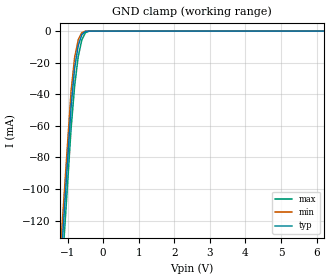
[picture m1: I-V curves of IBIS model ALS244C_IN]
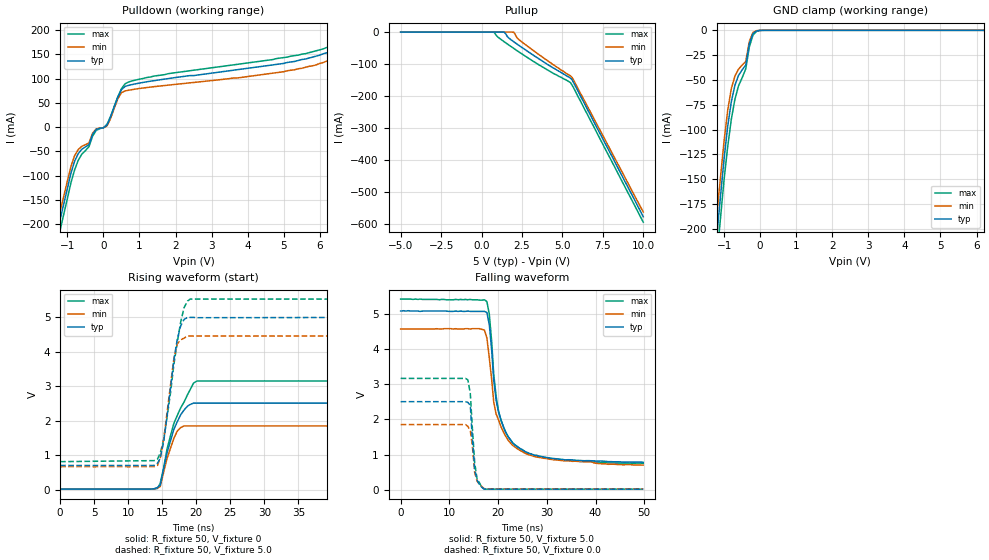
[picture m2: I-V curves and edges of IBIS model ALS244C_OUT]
| TEXAS INSTRUMENTS INCORPORATED
| Standard Linear and Logic Group
| IBIS Model of SN74ALS244C
| OCTAL BUFFERS AND LINE DRIVERS WITH 3-STATE OUTPUTS
| SOIC 20-pin (DW), SOP 20-pin (NS), SSOP 20-pin (DB), PDIP 20-pin (N) Package
[IBIS Ver]   3.2
[Comment Char]  |_char
[File Name]   sn54als244cw.ibs
[File Rev]   3.1
[Date]   Sept. 23, 2004
[Source]   Data created from Labo data at TI-SLL.
[Notes]   The following is an IBIS list for the ALS244C.
   - FILE REV HISTORY
   - 3.1 Re-Release IBIS file on 09/23/04
   - Power clamp data deleted as there is no power-clamp diode
|   Please contact sllibis@ti.com with questions and
|   comments concerning SLL IBIS models.
|   Modified for W ceramice package.  01/14/2009
[Disclaimer] Property of Texas Instruments Incorporated.  Unauthorized
   reproduction and/or distribution is strictly prohibited.
   This product is protected under copyright law.
   Created 2000, (C) Copyright 2000, Texas Instruments Inc.,
   All Rights Reserved.
   UNLESS THERE IS A SIGNED, WRITTEN AGREEMENT TO THE
   CONTRARY, TEXAS INSTRUMENTS () IS PROVIDING THE IBIS
   MODELS  AND WITHOUT ANY WARRANTY, EXPRESSED OR
   IMPLIED.  TI assumes no liability for:
   1) the accuracy of the IBIS models provided to your
   company;
   2) the proper functioning of these IBIS Models in your
   design or for any resulting applications; or
   3) infringement of patents, copyrights or intellectual
   property rights resulting from your use of these IBIS
   models.
   TI provides IBIS Models as a service to our customers.
   You and your company shall not distribute, sell or give
   these models to anyone else without prior written
   permission from TI.
   TI reserves the right to make changes to our products or
   to discontinue any semiconductor product or service
   without notice, and advises our customers to obtain the
   latest version of relevant information to verify, before
   placing orders, that the information being relied on is
   current.
   Please be aware that your receipt and use of the IBIS
   information provided shall serve as acceptance of these
   terms and conditions.  If you do not accept these terms,
   you should return or destroy the IBIS models and any
   other accompanying information immediately.
|   Component ALS244C_W
[Component]   ALS244C_W
[Manufacturer]  Texas Instruments, Inc.
[Package]
|   typ   min   max
R_pkg   0.134   0.093   0.180
L_pkg   6.136nH   4.282nH   8.371nH
C_pkg   1.657pF   1.224pF   2.253pF
[Pin]   signal_name   model_name   R_pin   L_pin   C_pin
1   1OE_NOT   ALS244C_IN   0.161   8.173nH   2.244pF
2   1A1   ALS244C_IN   0.163   7.152nH   2.034pF
3   2Y4   ALS244C_OUT   0.154   6.346nH   1.604pF
4   1A2   ALS244C_IN   0.093   4.737nH   1.272pF
5   2Y3   ALS244C_OUT   0.097   4.297nH   1.227pF
6   1A3   ALS244C_IN   0.096   4.289nH   1.226pF
7   2Y2   ALS244C_OUT   0.093   4.759nH   1.269pF
8   1A4   ALS244C_IN   0.143   6.181nH   1.554pF
9   2Y1   ALS244C_OUT   0.164   7.085nH   1.905pF
10   GND   GND   0.175   8.294nH   2.233pF
11   2A1   ALS244C_IN   0.180   8.371nH   2.239pF
12   1Y4   ALS244C_OUT   0.155   7.195nH   1.934pF
13   2A2   ALS244C_IN   0.154   6.339nH   1.581pF
14   1Y3   ALS244C_OUT   0.096   4.872nH   1.281pF
15   2A3   ALS244C_IN   0.097   4.338nH   1.233pF
16   1Y2   ALS244C_OUT   0.097   4.282nH   1.224pF
17   2A4   ALS244C_IN   0.093   4.726nH   1.262pF
18   1Y1   ALS244C_OUT   0.143   6.164nH   1.571pF
19   2OE_NOT   ALS244C_IN   0.159   6.938nH   2.001pF
20   VCC   POWER   0.166   8.186nH   2.253pF
| Models and submodels in the file (2): ALS244C_IN (Input), ALS244C_OUT (3-state)
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|   Model ALS244C_IN
[Model]   ALS244C_IN
Model_type  Input
Polarity   Non-Inverting
Vinl = 0.8
Vinh = 2.0
| variable   typ   min   max
C_comp   1.33pf   1.00pf   1.66pf
[Temperature Range]   25   0   70
[Voltage Range]   5.0   4.5   5.5
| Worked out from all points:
|   GND clamp passes 1 mA (typ) near -0.54 V on its own axis
[GND Clamp]
|   Voltage   I(typ)   I(min)   I(max)
-5V       -1.46A     -1.41A     -1.52A
-1.2V     -151mA     -138mA     -168mA
-1.1V     -117mA     -105mA     -132mA
-1V       -82.2mA    -71.2mA    -96.9mA
-900mV    -47.7mA    -37.7mA    -61.4mA
-800mV    -23.3mA    -16.5mA    -34.4mA
-700mV    -9.09mA    -5.49mA    -16.1mA
-600mV    -2.32mA    -965uA     -5.65mA
-500mV    -207uA     -49.9uA    -1.1mA
-400mV    -20.2uA    -16uA      -84.4uA
-300mV    -13.8uA    -14.7uA    -15.1uA
10V       2.13nA     225pA      4.62nA
|   Model ALS244C_OUT
[Model]   ALS244C_OUT
Model_type  3-state
Polarity   Non-Inverting
Enable   Active-Low
Vmeas = 2.5v
Cref = 15pf
| variable   typ   min   max
C_comp   5.8pf   4.35pf   7.25pf
[Temperature Range]   25   0   70
[Voltage Range]   5.0   4.5   5.5
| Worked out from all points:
|   slope of the pulldown table from 0 to 0.75 V, typ, clamps not added: 8.52 ohm
|   GND clamp passes 1 mA (typ) near -0.11 V on its own axis
|   rising waveform, R_fixture 50, V_fixture 0: 20-80 % time 2.21ns typ, 1.63ns min, 2.94ns max; typ from 0.021 V to 2.51 V
|   falling waveform, R_fixture 50, V_fixture 5.0: 20-80 % time 3.03ns typ, 3.61ns min, 2.9ns max; typ from 5.07 V to 0.782 V
|   rising waveform, R_fixture 50, V_fixture 5.0: 20-80 % time 1.7ns typ, 1.46ns min, 2.03ns max; typ from 0.706 V to 4.99 V
|   falling waveform, R_fixture 50, V_fixture 0.0: 20-80 % time 832ps typ, 914ps min, 943ps max; typ from 2.5 V to 0.019 V
[Pulldown]
|   Voltage   I(typ)   I(min)   I(max)
-5V       -1.4A      -1.34A     -1.44A
-1.4V     -254mA     -234mA     -276mA
-1.2V     -190mA     -173mA     -212mA
-900mV    -94.5mA    -80.4mA    -114mA
-700mV    -54.5mA    -46.1mA    -68.4mA
-200mV    -4.82mA    -3.55mA    -6.79mA
100mV     4.21mA     2.48mA     5.91mA
500mV     76.9mA     70.9mA     79.1mA
700mV     86mA       75.9mA     92.9mA
5.8V      144mA      126mA      155mA
7.6V      239mA      228mA      252mA
10V       425mA      436mA      450mA
[Pullup]
|   Voltage   I(typ)   I(min)   I(max)
-5V       18.8nA     1.71nA     273nA
700mV     18.8nA     1.71nA     -78.4uA
800mV     18.8nA     1.71nA     -1.62mA
1V        18.8nA     1.71nA     -15mA
1.4V      -389uA     1.71nA     -30.2mA
1.6V      -14.4mA    1.69nA     -37.3mA
2V        -30.5mA    -634uA     -51.3mA
2.2V      -37.6mA    -18.3mA    -58.2mA
2.6V      -51.7mA    -35mA      -71.7mA
5.5V      -144mA     -137mA     -158mA
5.7V      -159mA     -151mA     -175mA
10V       -578mA     -563mA     -595mA
[GND Clamp]
|   Voltage   I(typ)   I(min)   I(max)
-5V       -1.67A     -1.58A     -1.72A
-1.3V     -245mA     -222mA     -268mA
-1.2V     -206mA     -185mA     -228mA
-1.1V     -167mA     -148mA     -189mA
-900mV    -96.5mA    -80.3mA    -117mA
-800mV    -71.9mA    -58.7mA    -89.6mA
-600mV    -45.4mA    -39.1mA    -55.9mA
-400mV    -35mA      -31.3mA    -38.8mA
-300mV    -13.4mA    -11.1mA    -16.7mA
-200mV    -3.29mA    -2.13mA    -4.83mA
-100mV    -596uA     -308uA     -1.06mA
10V       3.02nA     210pA      25.3nA
[Ramp]
| variable   typ   min   max
dV/dt_r   1.52E+00/2.32E-09   1.31E+00/2.29E-09   1.70E+00/2.40E-09
dV/dt_f   2.63E+00/3.12E-09   2.33E+00/3.42E-09   2.86E+00/2.98E-09
R_load = 50
[Rising Waveform]
R_fixture = 50
V_fixture = 0
|   Time   V(typ)   V(min)   V(max)
0s        20.9mV     20.5mV     20.2mV
14.3ns    69.6mV     56.8mV     40.8mV
14.7ns    133mV      98.1mV     191mV
15.7ns    1.07V      908mV      1.18V
16.7ns    1.75V      1.49V      1.92V
17.2ns    1.97V      1.7V       2.15V
18.7ns    2.42V      1.85V      2.75V
19.6ns    2.51V      1.85V      3.09V
20.1ns    2.51V      1.85V      3.15V
49.8ns    2.51V      1.85V      3.15V
[Falling Waveform]
R_fixture = 50
V_fixture = 5.0
V_fixture_min = 4.5
V_fixture_max = 5.5
|   Time   V(typ)   V(min)   V(max)
0s        5.07V      4.56V      5.41V
16.2ns    5.06V      4.57V      5.38V
17.7ns    5.03V      4.31V      5.34V
18.2ns    4.68V      3.74V      4.98V
19.1ns    3.13V      2.5V       3.29V
20.1ns    2.2V       1.98V      2.23V
22.1ns    1.5V       1.4V       1.5V
25ns      1.14V      1.08V      1.12V
33.8ns    849mV      821mV      837mV
49.8ns    782mV      702mV      754mV
[Rising Waveform]
R_fixture = 50
V_fixture = 5.0
V_fixture_min = 4.5
V_fixture_max = 5.5
|   Time   V(typ)   V(min)   V(max)
0s        706mV      670mV      816mV
14.3ns    769mV      707mV      890mV
14.7ns    918mV      916mV      1.06V
15.2ns    1.39V      1.45V      1.45V
16.2ns    2.93V      3.01V      2.79V
16.7ns    3.75V      3.79V      3.62V
17.2ns    4.35V      4.22V      4.26V
18.2ns    4.93V      4.39V      5.27V
19.1ns    4.99V      4.45V      5.52V
49.8ns    4.99V      4.45V      5.52V
[Falling Waveform]
R_fixture = 50
V_fixture = 0.0
|   Time   V(typ)   V(min)   V(max)
0s        2.5V       1.85V      3.16V
13.3ns    2.5V       1.85V      3.16V
13.8ns    2.48V      1.8V       3.12V
14.3ns    2.39V      1.67V      2.73V
14.7ns    1.48V      1.27V      1.79V
15.2ns    577mV      488mV      767mV
15.7ns    273mV      246mV      299mV
16.7ns    67.1mV     89.5mV     58.3mV
17.2ns    19.2mV     27.6mV     19.2mV
49.8ns    19.2mV     27.6mV     19.2mV
